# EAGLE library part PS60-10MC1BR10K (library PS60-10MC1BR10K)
Slide Potentiometers 10K ohm 20% 60mm Slide Potentiometer Source: Datasheet
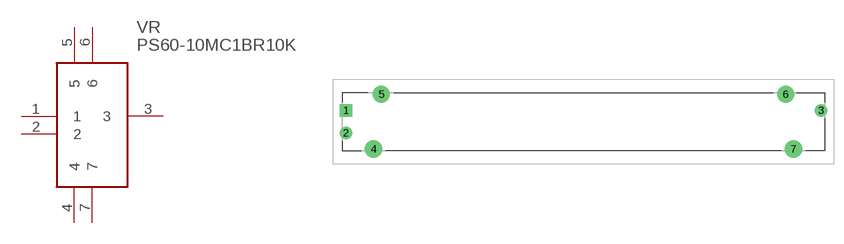
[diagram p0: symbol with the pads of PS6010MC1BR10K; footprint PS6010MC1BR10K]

Designator prefix VR

## PS60-10MC1BR10K (Description: Slide Potentiometers 10K ohm 20% 60mm Slide Potentiometer; Height: 15mm; Manufacturer_Name: TT Electronics; Manufacturer_Part_Number: PS60-10MC1BR10K; Mouser_Part_Number: 858-PS60-10MC1BR10K; Mouser_Price-Stock: https://www.mouser.co.uk/ProductDetail/BI-Technologies-TT-Electronics/PS60-10MC1BR10K?qs=INZo0Duj8JSwSdfUIJGnCA%3D%3D)  [PS6010MC1BR10K]
1  1
2  2
3  3
4  4
5  5
6  6
7  7

## Footprint PS6010MC1BR10K (pad centres in mm)
PS60-10MC1BR10K-1
drill 1.3 pad 1.95 square: 1 0,0
drill 1.3 pad 1.95: 2 0,-3.5; 3 73.8,0
drill 1.8 pad 2.7: 4 4.3,-6; 5 5.5,2.5; 6 68.3,2.5; 7 69.5,-6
